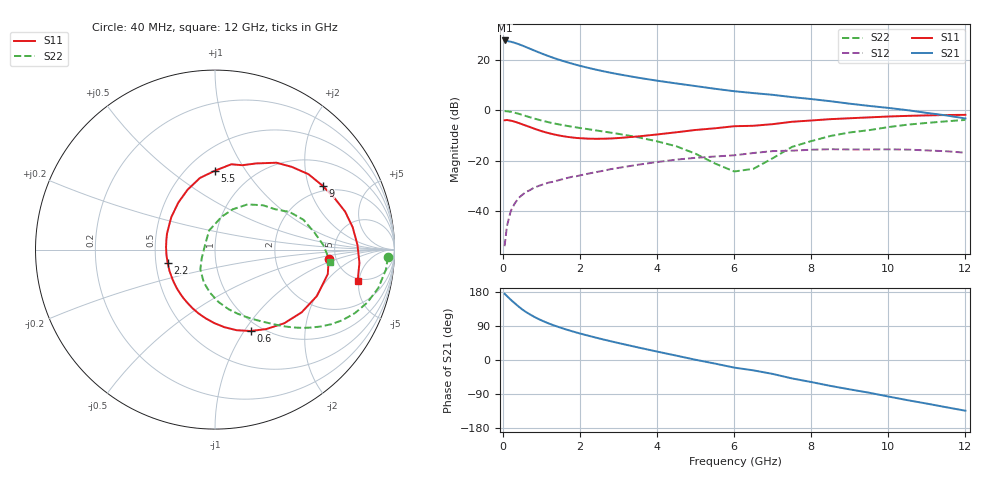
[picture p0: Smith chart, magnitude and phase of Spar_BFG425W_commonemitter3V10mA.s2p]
! Filename: 310bfg425.001
! BFG425W Field C1
! V1=8.398E-001V,V2=3.000E+000V, I1=1.270E-004A, I2=1.002E-002A
# GHz  S  MA  R 50
!  S11  S21  S12  S22
!Freq(GHz)  Mag  Ang  Mag  Ang  Mag  Ang  Mag  Ang
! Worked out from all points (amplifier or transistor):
!   44 points, 40 MHz to 12 GHz, reference 50 ohm
!   highest |S21| = 27.8 dB at 40 MHz (marker M1)
!   |S21| within 3 dB of that: start of sweep to 653 MHz
!   unconditionally stable (mu >= 1): 1.873 GHz to end of sweep
!   at 700 MHz: K = 0.53, MSG = 28.1 dB, |S12| = -31.7 dB
!   at 2.4 GHz: K = 1.11, MAG = 18.4 dB, |S12| = -24.6 dB
!   at 12 GHz: K = 1.40, MAG = 3.0 dB, |S12| = -16.8 dB
!   S11 on the Smith chart (normalised r, x): 40 MHz: 4.34, -0.79; 600 MHz: 0.89, -1.07; 2.2 GHz: 0.58, -0.09; 5.5 GHz: 0.68, +0.74; 9 GHz: 1.79, +2.48; 12 GHz: 4.63, -4.82
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0.04  0.636 -4.9  24.5 174.7  0.002 67.8  0.964 -2.5
0.2  0.624 -24.4  23.11 159.0  0.01 76.0  0.935 -13.2
0.3  0.596 -35.9  22 150.0  0.014 71.8  0.899 -19.1
0.4  0.563 -46.9  20.73 141.4  0.018 66.7  0.857 -24.3
0.5  0.527 -57.1  19.41 133.2  0.021 63.1  0.813 -28.9
0.6  0.495 -66.4  18.03 126.3  0.024 60.1  0.769 -32.7
0.8  0.435 -83.2  15.57 114.4  0.029 55.4  0.691 -38.9
0.9  0.409 -90.7  14.49 109.2  0.031 53.7  0.658 -41.5
1  0.386 -97.9  13.5 104.4  0.033 52.4  0.628 -43.8
1.2  0.35 -111.0  11.82 95.9  0.037 50.1  0.577 -47.8
1.4  0.323 -122.9  10.46 88.5  0.04 48.5  0.535 -51.3
1.6  0.303 -134.5  9.353 81.7  0.044 47.1  0.501 -54.5
2.2  0.274 -164.6  7.024 64.5  0.055 42.7  0.423 -63.8
3  0.282 161.4  5.21 44.7  0.072 35.4  0.341 -77.1
3.5  0.303 143.7  4.464 33.2  0.083 29.8  0.292 -86.3
4.5  0.367 114.6  3.425 11.5  0.105 16.6  0.193 -108.9
5.5  0.44 89.9  2.684 -9.4  0.121 2.0  0.088 -147.0
6.5  0.494 72.1  2.203 -27.4  0.142 -9.2  0.069 135.4
8.5  0.669 38.9  1.518 -68.4  0.169 -45.9  0.31 54.3
9  0.697 30.7  1.356 -77.6  0.167 -54.2  0.364 42.8
10.5  0.777 9.3  1.007 -106.1  0.166 -81.3  0.52 18.7
12  0.814 -12.4  0.69 -133.8  0.144 -111.7  0.646 -6.2
